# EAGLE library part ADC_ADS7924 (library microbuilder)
ADS7924 - 12-bit 4-Channel I2C ADC AVDD: 2.2-5.5V DVDD: 1.65V-5.5V Sampling Rate: 100ksps I2C Address: ADDR low = 1001000x, ADDR DVDD = 1001001x Digital Threshold Comparators The ADS794 is a relatively low-power device and can be useful in certain low-power scenarios since it can be configured to regularly check the voltage on the analog input pins, and throw an interrupt or pull an MCU out of reset when a specific condition is met. Each of the four inputs has it's own programmable threshold level. It could be used to monitor the input level of solar or other ambient energy sources, and when the level is sufficiently high, wakeup the MCU to perform read some sensor data, etc., or wait until a supercap is charged to a sufficiently high level before waking the MCU.
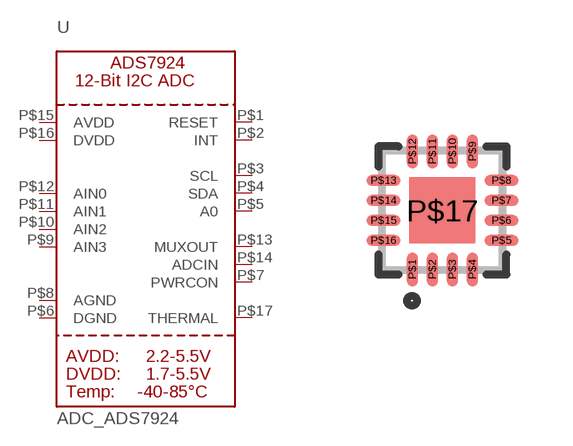
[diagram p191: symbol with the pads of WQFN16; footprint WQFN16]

Designator prefix U

## ADC_ADS7924  [WQFN16]
P$1  RESET
P$2  INT
P$3  SCL
P$4  SDA
P$5  A0
P$6  DGND
P$7  PWRCON
P$8  AGND
P$9  AIN3
P$10  AIN2
P$11  AIN1
P$12  AIN0
P$13  MUXOUT
P$14  ADCIN
P$15  AVDD
P$16  DVDD
P$17  THERMAL

## Footprint WQFN16 (pad centres in mm)
16-PWQFN 3.0x3.0mm Source: http://www.ti.com/lit/ds/symlink/ads7924.pdf
smd 0.28 x 0.85: P$1 -0.75,-1.475; P$2 -0.25,-1.475; P$3 0.25,-1.475; P$4 0.75,-1.475; P$9 0.75,1.475; P$10 0.25,1.475; P$11 -0.25,1.475; P$12 -0.75,1.475
smd 0.85 x 0.28: P$5 1.475,-0.75; P$6 1.475,-0.25; P$7 1.475,0.25; P$8 1.475,0.75; P$13 -1.475,0.75; P$14 -1.475,0.25; P$15 -1.475,-0.25; P$16 -1.475,-0.75
smd 1.65 x 1.65: P$17 0,0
